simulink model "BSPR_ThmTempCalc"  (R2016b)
settings: Solver=FixedStepDiscrete  StartTime=0.0  StopTime=10.0  FixedStep=0.02  RelTol=1e-3  EnableMultiTasking=on
undefined symbols (not defined in the file): BSPR_cofClntTempFlt_C, BSPR_tClntDsTInitVal_C, BSPR_tClntDsTLoLim_C, BSPR_tClntDsTUpLim_C, BSPR_tClntUsTInitVal_C, BSPR_tClntUsTLoLim_C, BSPR_tClntUsTUpLim_C, BSPR_tCoolant_CUR, BSPR_tCoolant_CUR_X, BSPR_uClntDsTInitVal_C, BSPR_uClntUsTInitVal_C

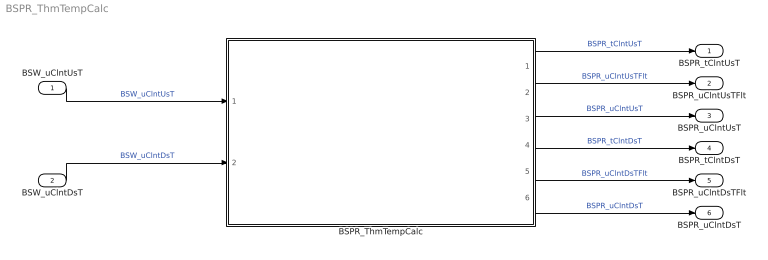
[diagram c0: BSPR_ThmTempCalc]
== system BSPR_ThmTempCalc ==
  BSW_uClntUsT : Inport
  BSW_uClntDsT : Inport  Port=2
  BSPR_ThmTempCalc : Subsystem
  BSPR_tClntUsT : Outport  OutDataTypeStr=single
  BSPR_uClntUsTFlt : Outport  Port=2  OutDataTypeStr=single
  BSPR_uClntUsT : Outport  Port=3  OutDataTypeStr=single
  BSPR_tClntDsT : Outport  Port=4  OutDataTypeStr=single
  BSPR_uClntDsTFlt : Outport  Port=5  OutDataTypeStr=single
  BSPR_uClntDsT : Outport  Port=6  OutDataTypeStr=single
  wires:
  BSW_uClntDsT/1 -> BSPR_ThmTempCalc/2(BSW_uClntDsT)  "BSW_uClntDsT"
  BSW_uClntUsT/1 -> BSPR_ThmTempCalc/1(BSW_uClntUsT)  "BSW_uClntUsT"
  BSPR_ThmTempCalc/1(BSPR_tClntUsT) -> BSPR_tClntUsT/1  "BSPR_tClntUsT"
  BSPR_ThmTempCalc/2(BSPR_uClntUsTFlt) -> BSPR_uClntUsTFlt/1  "BSPR_uClntUsTFlt"
  BSPR_ThmTempCalc/3(BSPR_uClntUsT) -> BSPR_uClntUsT/1  "BSPR_uClntUsT"
  BSPR_ThmTempCalc/4(BSPR_tClntDsT) -> BSPR_tClntDsT/1  "BSPR_tClntDsT"
  BSPR_ThmTempCalc/5(BSPR_uClntDsTFlt) -> BSPR_uClntDsTFlt/1  "BSPR_uClntDsTFlt"
  BSPR_ThmTempCalc/6(BSPR_uClntDsT) -> BSPR_uClntDsT/1  "BSPR_uClntDsT"

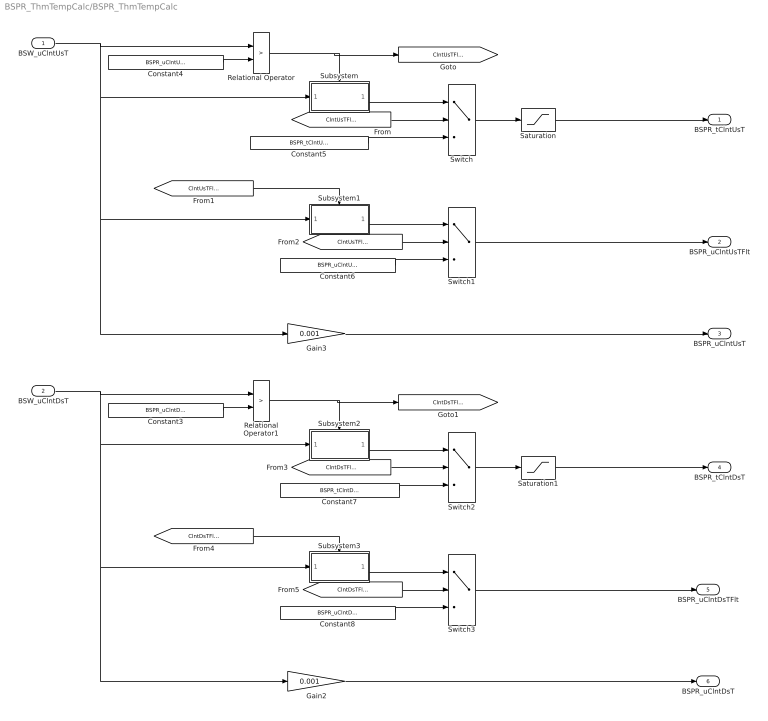
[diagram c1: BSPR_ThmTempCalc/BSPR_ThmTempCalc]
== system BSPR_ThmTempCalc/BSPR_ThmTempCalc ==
  BSW_uClntUsT : Inport
  BSW_uClntDsT : Inport  Port=2
  Constant3 : Constant  Value=BSPR_uClntDsTInitVal_C  OutDataTypeStr=single
  Constant4 : Constant  Value=BSPR_uClntUsTInitVal_C  OutDataTypeStr=single
  Constant5 : Constant  Value=BSPR_tClntUsTInitVal_C  OutDataTypeStr=single
  Constant6 : Constant  Value=BSPR_uClntUsTInitVal_C  OutDataTypeStr=single
  Constant7 : Constant  Value=BSPR_tClntDsTInitVal_C  OutDataTypeStr=single
  Constant8 : Constant  Value=BSPR_uClntDsTInitVal_C  OutDataTypeStr=single
  Gain2 : Gain  Gain=0.001
  Gain3 : Gain  Gain=0.001
  Relational Operator : RelationalOperator  Operator=>  OutDataTypeStr=boolean  RndMeth=Simplest
  Relational Operator1 : RelationalOperator  Operator=>  OutDataTypeStr=boolean  RndMeth=Simplest
  Saturation : Saturate  UpperLimit=BSPR_tClntUsTUpLim_C  LowerLimit=BSPR_tClntUsTLoLim_C
  Saturation1 : Saturate  UpperLimit=BSPR_tClntDsTUpLim_C  LowerLimit=BSPR_tClntDsTLoLim_C
  Subsystem : Subsystem
  Subsystem1 : Subsystem
  Subsystem2 : Subsystem
  Subsystem3 : Subsystem
  Switch{,1..3} (4 alike) : Switch  Criteria=u2 ~= 0
  BSPR_tClntUsT : Outport  OutDataTypeStr=single
  BSPR_uClntUsTFlt : Outport  Port=2  OutDataTypeStr=single
  BSPR_uClntUsT : Outport  Port=3  OutDataTypeStr=single
  BSPR_tClntDsT : Outport  Port=4  OutDataTypeStr=single
  BSPR_uClntDsTFlt : Outport  Port=5  OutDataTypeStr=single
  BSPR_uClntDsT : Outport  Port=6  OutDataTypeStr=single
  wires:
  Switch/1 -> Saturation/1
  Subsystem/1(tTemp) -> Switch/1
  Relational Operator/1 -> [ClntUsTFltEna], Subsystem/Enable
  Constant4/1 -> Relational Operator/2
  Constant5/1 -> Switch/3
  Gain3/1 -> BSPR_uClntUsT/1
  Saturation/1 -> BSPR_tClntUsT/1
  Switch1/1 -> BSPR_uClntUsTFlt/1
  Constant6/1 -> Switch1/3
  Subsystem1/1(uTemp) -> Switch1/1
  [ClntUsTFltEna] -> Switch/2
  [ClntUsTFltEna] -> Subsystem1/Enable
  BSW_uClntUsT/1 -> Subsystem1/1(u), Gain3/1, Subsystem/1(u), Relational Operator/1
  [ClntUsTFltEna] -> Switch1/2
  Switch2/1 -> Saturation1/1
  Subsystem2/1(tTemp) -> Switch2/1
  Relational Operator1/1 -> Subsystem2/Enable, [ClntDsTFltEna]
  Constant3/1 -> Relational Operator1/2
  Constant7/1 -> Switch2/3
  Gain2/1 -> BSPR_uClntDsT/1
  Saturation1/1 -> BSPR_tClntDsT/1
  Switch3/1 -> BSPR_uClntDsTFlt/1
  Constant8/1 -> Switch3/3
  Subsystem3/1(uTemp) -> Switch3/1
  [ClntDsTFltEna] -> Switch2/2
  [ClntDsTFltEna] -> Subsystem3/Enable
  BSW_uClntDsT/1 -> Relational Operator1/1, Subsystem2/1(u), Gain2/1, Subsystem3/1(u)
  [ClntDsTFltEna] -> Switch3/2

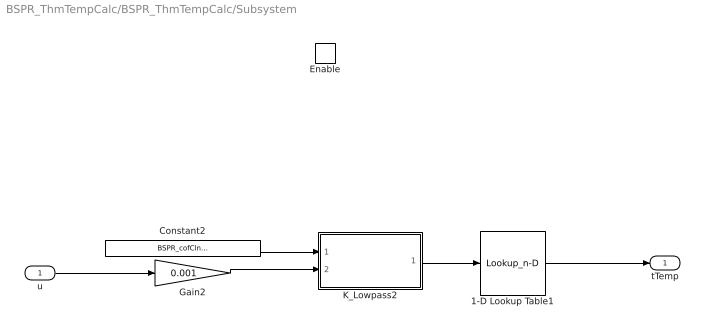
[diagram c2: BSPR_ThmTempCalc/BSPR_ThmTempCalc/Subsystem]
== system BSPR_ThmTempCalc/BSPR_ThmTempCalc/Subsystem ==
  u : Inport  OutDataTypeStr=single
  Enable : EnablePort  StatesWhenEnabling=reset
  1-D Lookup Table1 : Lookup_n-D  NumberOfTableDimensions=1  BreakpointsForDimension1=BSPR_tCoolant_CUR_X  Table=BSPR_tCoolant_CUR  ExtrapMethod=Clip  InternalRulePriority=Speed  RndMeth=Simplest
  Constant2 : Constant  Value=BSPR_cofClntTempFlt_C  OutDataTypeStr=single
  Gain2 : Gain  Gain=0.001
  K_Lowpass2 : Subsystem  TreatAsAtomicUnit=on  RTWFcnName=K_Lowpass  RTWFileName=SrvLib
  tTemp : Outport  OutDataTypeStr=single
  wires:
  K_Lowpass2/1(y) -> 1-D Lookup Table1/1
  Constant2/1 -> K_Lowpass2/1(k)
  u/1 -> Gain2/1
  1-D Lookup Table1/1 -> tTemp/1
  Gain2/1 -> K_Lowpass2/2(u)

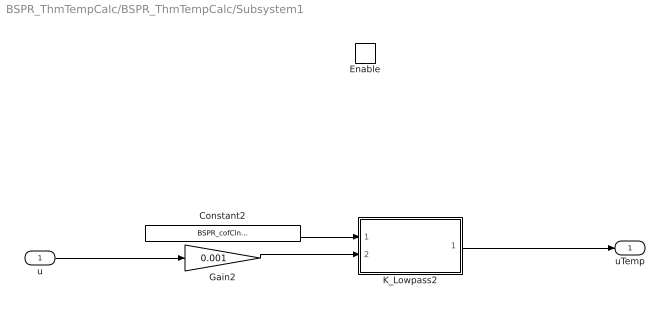
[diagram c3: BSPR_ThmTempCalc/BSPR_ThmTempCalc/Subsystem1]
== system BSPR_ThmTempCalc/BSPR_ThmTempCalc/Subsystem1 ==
  u : Inport  OutDataTypeStr=single
  Enable : EnablePort  StatesWhenEnabling=reset
  Constant2 : Constant  Value=BSPR_cofClntTempFlt_C  OutDataTypeStr=single
  Gain2 : Gain  Gain=0.001
  K_Lowpass2 : Subsystem  TreatAsAtomicUnit=on  RTWFcnName=K_Lowpass  RTWFileName=SrvLib
  uTemp : Outport  OutDataTypeStr=single
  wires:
  u/1 -> Gain2/1
  Constant2/1 -> K_Lowpass2/1(k)
  Gain2/1 -> K_Lowpass2/2(u)
  K_Lowpass2/1(y) -> uTemp/1

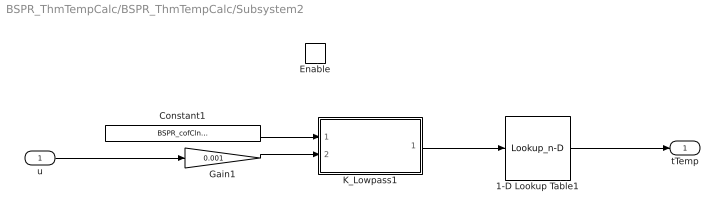
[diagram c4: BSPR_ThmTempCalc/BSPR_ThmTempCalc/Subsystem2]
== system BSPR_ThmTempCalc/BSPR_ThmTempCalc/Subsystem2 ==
  u : Inport  OutDataTypeStr=single
  Enable : EnablePort  StatesWhenEnabling=reset
  1-D Lookup Table1 : Lookup_n-D  NumberOfTableDimensions=1  BreakpointsForDimension1=BSPR_tCoolant_CUR_X  Table=BSPR_tCoolant_CUR  ExtrapMethod=Clip  InternalRulePriority=Speed  RndMeth=Simplest
  Constant1 : Constant  Value=BSPR_cofClntTempFlt_C  OutDataTypeStr=single
  Gain1 : Gain  Gain=0.001
  K_Lowpass1 : Subsystem  TreatAsAtomicUnit=on  RTWFcnName=K_Lowpass  RTWFileName=SrvLib
  tTemp : Outport  OutDataTypeStr=single
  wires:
  u/1 -> Gain1/1
  K_Lowpass1/1(y) -> 1-D Lookup Table1/1
  Constant1/1 -> K_Lowpass1/1(k)
  Gain1/1 -> K_Lowpass1/2(u)
  1-D Lookup Table1/1 -> tTemp/1

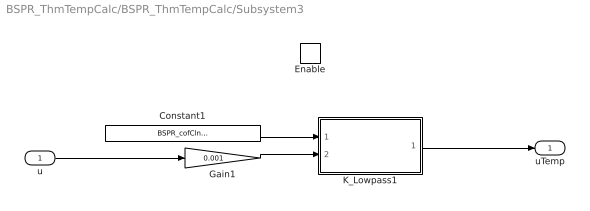
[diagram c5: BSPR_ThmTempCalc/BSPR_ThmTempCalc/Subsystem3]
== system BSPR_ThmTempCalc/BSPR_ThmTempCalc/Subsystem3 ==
  u : Inport  OutDataTypeStr=single
  Enable : EnablePort  StatesWhenEnabling=reset
  Constant1 : Constant  Value=BSPR_cofClntTempFlt_C  OutDataTypeStr=single
  Gain1 : Gain  Gain=0.001
  K_Lowpass1 : Subsystem  TreatAsAtomicUnit=on  RTWFcnName=K_Lowpass  RTWFileName=SrvLib
  uTemp : Outport  OutDataTypeStr=single
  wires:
  u/1 -> Gain1/1
  Constant1/1 -> K_Lowpass1/1(k)
  Gain1/1 -> K_Lowpass1/2(u)
  K_Lowpass1/1(y) -> uTemp/1

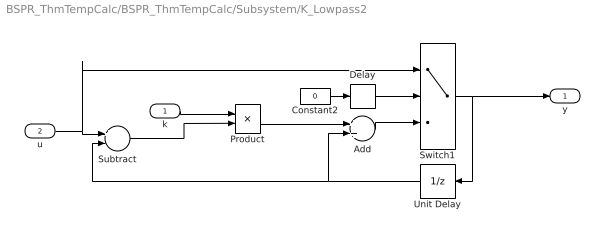
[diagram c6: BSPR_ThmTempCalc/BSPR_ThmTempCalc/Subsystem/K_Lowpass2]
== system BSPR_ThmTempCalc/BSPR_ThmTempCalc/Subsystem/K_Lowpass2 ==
  k : Inport
  u : Inport  Port=2
  Add : Sum
  Constant2 : Constant  Value=0
  Delay : Delay  DelayLength=1  InitialCondition=1
  Product : Product
  Subtract : Sum  Inputs=+-
  Switch1 : Switch  Criteria=u2 > Threshold
  Unit Delay : UnitDelay  SampleTime=-1
  y : Outport
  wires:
  k/1 -> Product/1
  Product/1 -> Add/1
  Constant2/1 -> Delay/1
  Unit Delay/1 -> Subtract/2, Add/2
  Subtract/1 -> Product/2
  Add/1 -> Switch1/3
  Delay/1 -> Switch1/2
  Switch1/1 -> y/1, Unit Delay/1
  u/1 -> Switch1/1, Subtract/1

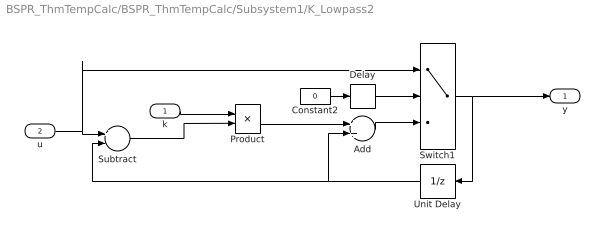
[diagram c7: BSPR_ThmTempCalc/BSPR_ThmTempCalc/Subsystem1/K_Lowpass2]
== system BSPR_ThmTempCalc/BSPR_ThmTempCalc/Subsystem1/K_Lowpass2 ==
  k : Inport
  u : Inport  Port=2
  Add : Sum
  Constant2 : Constant  Value=0
  Delay : Delay  DelayLength=1  InitialCondition=1
  Product : Product
  Subtract : Sum  Inputs=+-
  Switch1 : Switch  Criteria=u2 > Threshold
  Unit Delay : UnitDelay  SampleTime=-1
  y : Outport
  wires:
  k/1 -> Product/1
  Product/1 -> Add/1
  Constant2/1 -> Delay/1
  Unit Delay/1 -> Subtract/2, Add/2
  Subtract/1 -> Product/2
  Add/1 -> Switch1/3
  Delay/1 -> Switch1/2
  Switch1/1 -> y/1, Unit Delay/1
  u/1 -> Switch1/1, Subtract/1

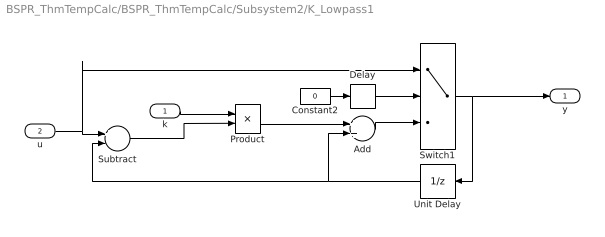
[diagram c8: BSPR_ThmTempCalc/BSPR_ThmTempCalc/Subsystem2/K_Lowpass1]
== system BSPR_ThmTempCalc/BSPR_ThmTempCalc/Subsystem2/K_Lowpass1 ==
  k : Inport
  u : Inport  Port=2
  Add : Sum
  Constant2 : Constant  Value=0
  Delay : Delay  DelayLength=1  InitialCondition=1
  Product : Product
  Subtract : Sum  Inputs=+-
  Switch1 : Switch  Criteria=u2 > Threshold
  Unit Delay : UnitDelay  SampleTime=-1
  y : Outport
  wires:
  u/1 -> Subtract/1, Switch1/1
  Switch1/1 -> Unit Delay/1, y/1
  Delay/1 -> Switch1/2
  Add/1 -> Switch1/3
  Subtract/1 -> Product/2
  Unit Delay/1 -> Add/2, Subtract/2
  Constant2/1 -> Delay/1
  Product/1 -> Add/1
  k/1 -> Product/1

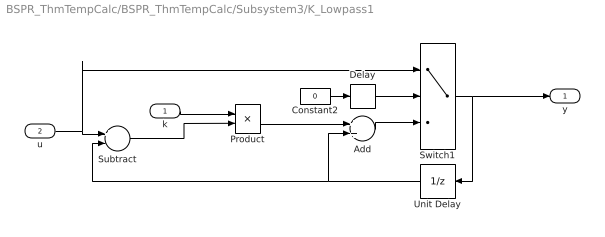
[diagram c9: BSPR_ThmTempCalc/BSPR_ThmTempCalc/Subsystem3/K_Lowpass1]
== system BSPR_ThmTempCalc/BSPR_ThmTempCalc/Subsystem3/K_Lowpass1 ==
  k : Inport
  u : Inport  Port=2
  Add : Sum
  Constant2 : Constant  Value=0
  Delay : Delay  DelayLength=1  InitialCondition=1
  Product : Product
  Subtract : Sum  Inputs=+-
  Switch1 : Switch  Criteria=u2 > Threshold
  Unit Delay : UnitDelay  SampleTime=-1
  y : Outport
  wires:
  u/1 -> Subtract/1, Switch1/1
  Switch1/1 -> Unit Delay/1, y/1
  Delay/1 -> Switch1/2
  Add/1 -> Switch1/3
  Subtract/1 -> Product/2
  Unit Delay/1 -> Add/2, Subtract/2
  Constant2/1 -> Delay/1
  Product/1 -> Add/1
  k/1 -> Product/1
